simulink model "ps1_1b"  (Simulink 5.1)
settings: Solver=ode45  StartTime=0.0  StopTime=10.0  RelTol=1e-3
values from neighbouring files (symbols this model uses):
  d = 0.0001    [ps4_3.m]
  s = tf('s')    [ps7_3_2.m]    (also in ps4_2.m; ps7_1_2.m; ps4_3.m; ps2_3.m)
libraries: cstblocks x3

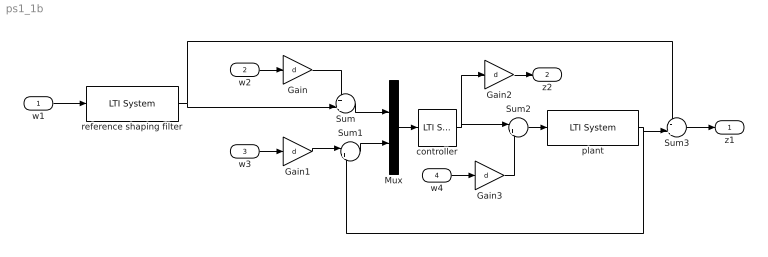
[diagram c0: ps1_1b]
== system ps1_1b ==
  w1 : Inport
  w2 : Inport  Port=2
  w3 : Inport  Port=3
  w4 : Inport  Port=4
  Gain{,1..3} (4 alike) : Gain  Gain=d
  Mux : Mux  Inputs=2
  Sum : Sum  Inputs=++|
  Sum1 : Sum  Inputs=|++
  Sum2 : Sum  Inputs=|++
  Sum3 : Sum  Inputs=-+|
  controller : cstblocks/LTI System  sys=K  IC=[]
  plant : cstblocks/LTI System  sys=s/(s^2+1)  IC=[]
  reference shaping filter : cstblocks/LTI System  sys=10/(s+10)  IC=[]
  z1 : Outport
  z2 : Outport  Port=2
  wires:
  w1/1 -> reference shaping filter/1
  w2/1 -> Gain/1
  Gain/1 -> Sum/1
  reference shaping filter/1 -> Sum/2, Sum3/1
  Gain1/1 -> Sum1/1
  w3/1 -> Gain1/1
  Gain2/1 -> z2/1
  Sum2/1 -> plant/1
  plant/1 -> Sum3/2, Sum1/2
  Sum3/1 -> z1/1
  Sum/1 -> Mux/1
  Sum1/1 -> Mux/2
  w4/1 -> Gain3/1
  controller/1 -> Sum2/1, Gain2/1
  Gain3/1 -> Sum2/2
  Mux/1 -> controller/1
